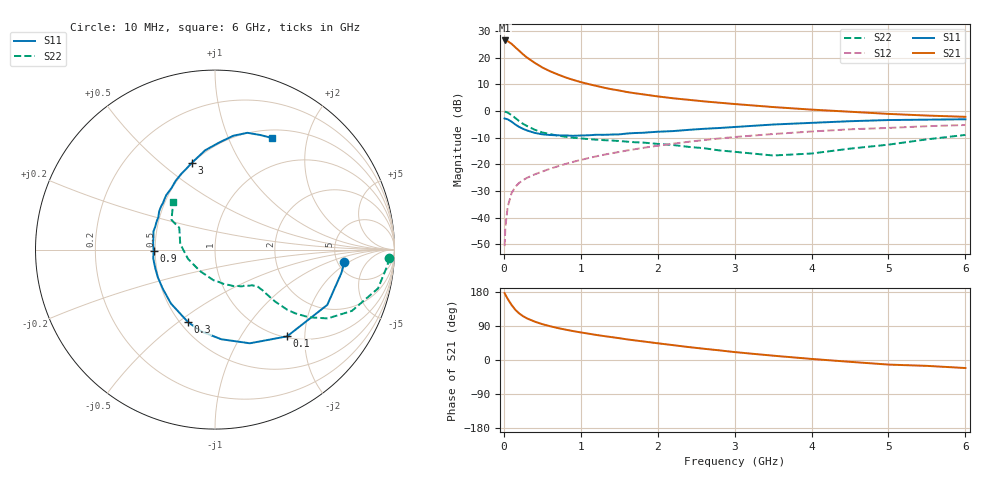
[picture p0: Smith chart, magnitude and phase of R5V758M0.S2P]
! SIEMENS Small Signal Semiconductors
! BFR183
! Si NPN RF Bipolar Junction Transistor in SOT23
! VCE = 0.75 V  IC = 8 mA
! Common Emitter S-Parameters:  May  1996
# GHz  S  MA  R  50
!  f  S11  S21  S12  S22
! GHz  MAG  ANG  MAG  ANG  MAG  ANG  MAG  ANG
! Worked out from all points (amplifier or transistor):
!   36 points, 10 MHz to 6 GHz, reference 50 ohm
!   highest |S21| = 26.5 dB at 10 MHz (marker M1)
!   |S21| within 3 dB of that: start of sweep to 165.6 MHz
!   unconditionally stable (mu >= 1): 766.3 MHz to 2.941 GHz
!   at 250 MHz: K = 0.57, MSG = 23.6 dB, |S12| = -26.0 dB
!   at 1.4 GHz: K = 1.08, MAG = 10.3 dB, |S12| = -15.9 dB
!   at 6 GHz: K = 0.95, MSG = 1.5 dB, |S12| = -5.3 dB
!   S11 on the Smith chart (normalised r, x): 10 MHz: 5.73, -1.70; 100 MHz: 1.02, -1.63; 300 MHz: 0.55, -0.54; 900 MHz: 0.49, -0.01; 3 GHz: 0.50, +0.64; 6 GHz: 0.60, +1.45
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0.01  0.7243 -5.6  21.05 176.4  0.0029 84.0  0.973 -2.7
0.02  0.7159 -10.6  20.79 172.3  0.0066 84.1  0.9639 -5.4
0.05  0.6974 -26.2  20.41 161.3  0.0159 77.9  0.9336 -13.4
0.1  0.6284 -50.3  18.22 145.4  0.0286 67.9  0.8359 -24.1
0.15  0.5569 -69.6  15.61 132.3  0.0378 61.8  0.7359 -31.4
0.2  0.5004 -86.1  13.46 122.8  0.0448 58.4  0.6446 -35.8
0.25  0.4616 -99.7  11.54 115.6  0.0503 56.6  0.5731 -38.4
0.3  0.431 -110.4  10.09 109.9  0.0555 56.4  0.5221 -39.8
0.4  0.388 -129.3  8.024 101.4  0.0644 56.3  0.4449 -40.8
0.5  0.3639 -142.8  6.55 94.6  0.073 57.2  0.395 -40.8
0.6  0.3543 -153.7  5.567 89.2  0.0822 57.9  0.3671 -40.7
0.7  0.3485 -162.9  4.853 84.4  0.0912 58.7  0.3458 -40.6
0.9  0.3418 -179.0  3.834 76.3  0.1109 59.4  0.3145 -40.9
1.1  0.3493 169.3  3.198 69.5  0.1305 59.4  0.2969 -42.7
1.3  0.3566 159.0  2.739 63.2  0.1508 58.5  0.2832 -44.7
1.6  0.3772 145.6  2.269 54.5  0.1811 56.8  0.2656 -49.4
2.2  0.419 125.6  1.73 39.2  0.2432 51.4  0.2297 -62.5
3  0.4999 105.1  1.35 20.9  0.3244 41.9  0.1712 -92.7
3.5  0.5563 95.6  1.184 11.4  0.3691 35.2  0.1459 -124.9
4.5  0.6422 80.9  0.967 -4.8  0.4528 22.1  0.1962 170.8
5.5  0.6867 68.3  0.82 -15.5  0.5173 10.4  0.2932 145.7
6  0.6976 63.1  0.776 -21.2  0.5454 2.8  0.355 131.0
